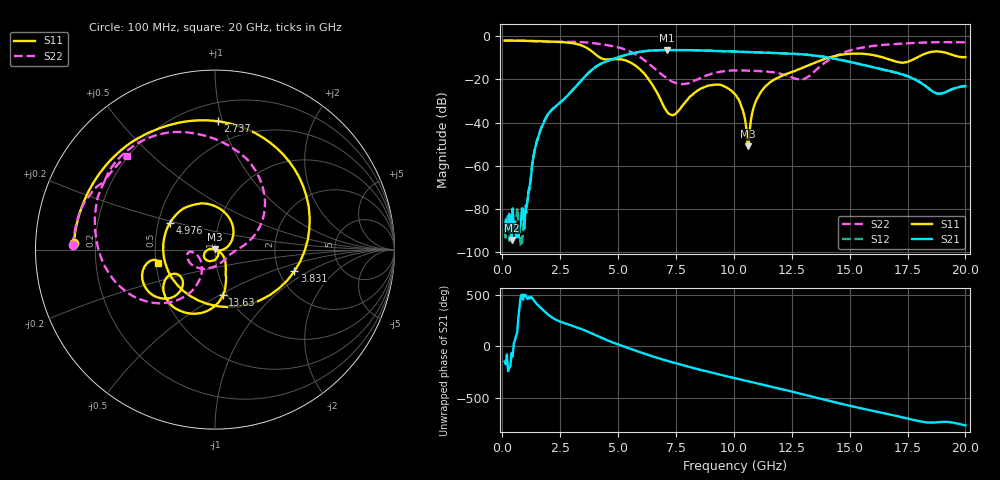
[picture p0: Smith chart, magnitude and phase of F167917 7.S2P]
!  2-Port S-parameters saved by WinCal
! VAR MeasName=S-Parameters (CALIBRATED_DATA) read from VNA (N5242A)
! VAR MeasDate=2016-11-22 9:00:00
! VAR NAME=F167917 7
! VAR FILENAME=F167917 7.S2P
! VAR DATE=2016-11-22 9:00:00
! VAR PHYS_PORTS=1,2
# Hz S DB R 50
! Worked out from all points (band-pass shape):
!   401 points, 100 MHz to 20 GHz, reference 50 ohm
!   highest |S21| = -6.44 dB at 7.115 GHz (marker M1); lowest = -94.3 dB at 398.5 MHz (marker M2)
!   |S21| within 3 dB of the highest: 5.114 GHz to 13.8 GHz (8.684 GHz wide, 91.8 % of centre)
!   lowest |S11| = -50.9 dB at 10.6 GHz (marker M3), VSWR 1.01, Z = 49.8 + j0.213 ohm
!   |S11| at or under -10 dB: 4.226 GHz to 14.09 GHz (9.864 GHz wide, 108 % of centre); 16.48 GHz to 17.9 GHz (1.417 GHz wide, 8.24 % of centre)
!   |S22| runs from -22.2 to -2.0 dB; largest |S21 - S12| = 0.0043
!   S11 on the Smith chart (normalised r, x): 100 MHz: 0.12, +0.02; 2.737 GHz: 0.33, +0.97; 3.831 GHz: 2.43, -0.74; 4.976 GHz: 0.58, +0.19; 13.63 GHz: 0.95, -0.52; 20 GHz: 0.51, -0.08
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1e8  -2.09 177.3  -90.36 -148.1  -90.33 -75.5  -2.03 178.3
3.985e8  -2.12 169.4  -94.27 -64.1  -92.39 4.5  -2.05 173.4
9.955e8  -2.22 153.3  -81.59 137.1  -78.50 128.7  -2.16 163.4
1.64225e9  -2.36 134.0  -43.82 14.5  -43.69 13.6  -2.51 152.7
2.73675e9  -2.91 88.7  -28.39 -140.9  -28.41 -141.4  -2.63 136.2
3.43325e9  -4.38 35.5  -20.29 165.0  -20.31 165.0  -2.81 120.5
3.83125e9  -6.77 -15.3  -15.97 127.6  -15.96 127.6  -3.15 109.9
4.22925e9  -10.02 -87.9  -12.98 86.8  -12.94 86.8  -3.71 98.9
4.9755e9  -10.70 149.1  -9.94 20.1  -9.91 19.6  -5.15 75.1
5.92075e9  -15.12 57.8  -7.31 -55.0  -7.33 -55.1  -9.52 35.5
6.7665e9  -27.92 -2.5  -6.50 -117.3  -6.51 -117.4  -16.75 4.9
7.11475e9  -34.88 -11.5  -6.44 -140.6  -6.45 -140.6  -19.56 -7.0
8.90575e9  -22.91 -116.0  -6.78 112.5  -6.76 112.5  -17.88 -123.5
1.005e10  -26.89 -174.0  -7.17 51.0  -7.18 51.1  -15.90 -159.1
1.059725e10  -50.90 131.6  -7.38 22.5  -7.39 22.5  -15.97 -167.2
1.09455e10  -30.25 -24.6  -7.53 4.3  -7.52 4.4  -16.10 -169.9
1.13435e10  -23.52 -40.9  -7.66 -16.6  -7.66 -16.3  -16.32 -172.8
1.338325e10  -12.83 -75.9  -8.87 -126.7  -8.83 -126.2  -17.27 -122.2
1.3632e10  -11.74 -80.3  -9.20 -140.6  -9.14 -140.2  -14.90 -117.3
1.67165e10  -10.81 -150.7  -16.13 61.6  -16.12 61.6  -3.85 -177.7
1.8806e10  -7.10 -154.3  -26.71 -14.2  -26.50 -14.3  -2.82 148.9
2e10  -9.74 -166.9  -23.17 -45.3  -23.04 -45.7  -2.88 133.2
